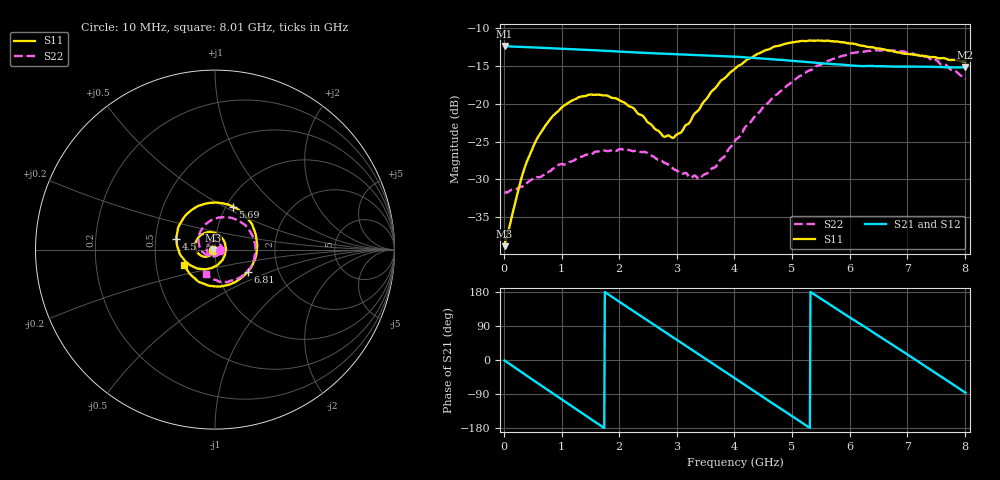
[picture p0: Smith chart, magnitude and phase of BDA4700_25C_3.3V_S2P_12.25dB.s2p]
!Agilent Technologies,E5071B,MY42404982,A.09.10
!Date: Mon Oct 20 18:08:10 2025
!Data & Calibration Information:
!Freq	S11:SOLT2(ON)	S21:SOLT2(ON)	S12:SOLT2(ON)	S22:SOLT2(ON)
# Hz S RI R 50
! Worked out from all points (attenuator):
!   801 points, 10 MHz to 8.01 GHz, reference 50 ohm
!   highest |S21| = -12.35 dB at 10 MHz (marker M1); lowest = -15.2 dB at 8 GHz (marker M2)
!   lowest |S11| = -38.8 dB at 10 MHz (marker M3), VSWR 1.02, Z = 48.9 - j0.167 ohm
!   |S11| at or under -10 dB: start of sweep to end of sweep
!   |S22| runs from -31.8 to -12.9 dB; largest |S21 - S12| = 0.0028
!   S11 on the Smith chart (normalised r, x): 10 MHz: 0.98, -0.00; 4.5 GHz: 0.64, +0.08; 5.69 GHz: 1.07, +0.55; 6.81 GHz: 1.39, -0.36; 8.01 GHz: 0.70, -0.12
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1e7  -0.0113 -0.00171  0.2412 -0.00522  0.2411 -0.00548  0.0261 -0.000946
3.3e8  -0.0223 -0.027  0.1952 -0.1354  0.1952 -0.1355  0.0228 -0.0171
5.6e8  -0.0424 -0.0391  0.123 -0.2009  0.1229 -0.2011  0.0144 -0.0294
8.7e8  -0.0775 -0.0345  -0.0021 -0.2329  -0.00199 -0.233  -0.00919 -0.0365
1.35e9  -0.11 0.0213  -0.1745 -0.1473  -0.1744 -0.1476  -0.0424 -0.0142
1.94e9  -0.0544 0.0942  -0.2089 0.0759  -0.2091 0.076  -0.0321 0.0367
2.33e9  0.0133 0.0848  -0.1111 0.1878  -0.1113 0.1878  0.000854 0.0486
2.68e9  0.0553 0.0364  0.0173 0.2146  0.0169 0.2144  0.0281 0.0322
2.95e9  0.0573 -0.0183  0.1119 0.1813  0.1116 0.1808  0.0355 0.00998
3.39e9  -4.5e-06 -0.0922  0.2032 0.0513  0.2036 0.0514  0.0183 -0.0261
3.67e9  -0.0666 -0.1085  0.2013 -0.0501  0.2014 -0.0507  -0.00823 -0.0373
4.01e9  -0.1531 -0.0755  0.1361 -0.1533  0.1364 -0.1529  -0.0482 -0.0301
4.5e9  -0.215 0.0581  -0.0277 -0.1972  -0.0273 -0.1976  -0.0899 0.0298
4.95e9  -0.1577 0.1974  -0.1549 -0.1155  -0.1545 -0.1164  -0.0747 0.1124
5.35e9  -0.0278 0.2602  -0.1875 0.0108  -0.1875 0.00975  -0.00453 0.1687
5.69e9  0.098 0.2397  -0.1468 0.1098  -0.1466 0.11  0.0824 0.1789
6.21e9  0.2243 0.0923  -0.00809 0.1776  -0.00573 0.1781  0.1985 0.0968
6.68e9  0.2098 -0.0827  0.1221 0.1277  0.1226 0.1275  0.2215 -0.0321
6.81e9  0.1814 -0.1236  0.1469 0.0974  0.1476 0.0964  0.2124 -0.0676
7.36e9  0.00355 -0.2049  0.1642 -0.0631  0.1642 -0.0633  0.1081 -0.1725
8e9  -0.1704 -0.0874  0.0141 -0.1735  0.0143 -0.1737  -0.0503 -0.1385
8.01e9  -0.1718 -0.0849  0.0109 -0.1737  0.0116 -0.1737  -0.0521 -0.1365
